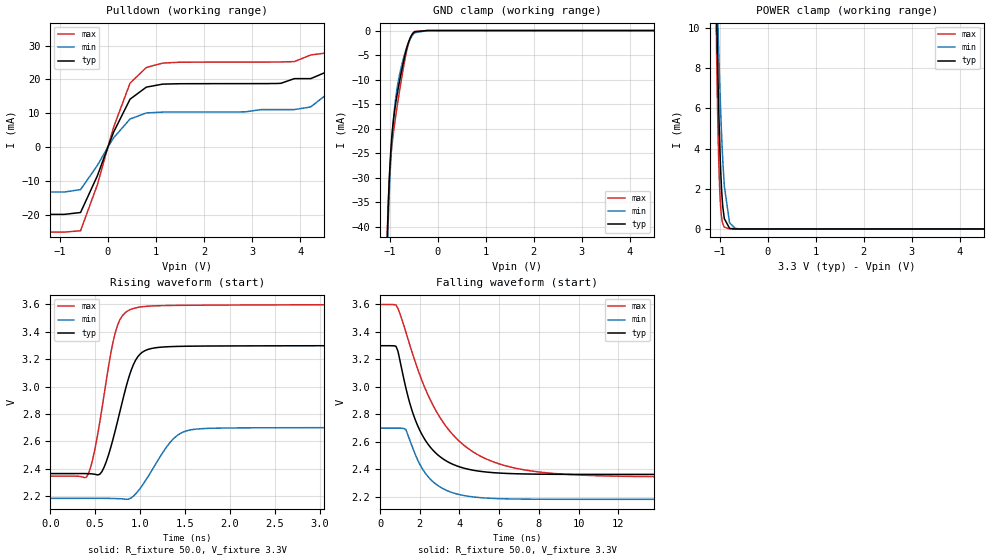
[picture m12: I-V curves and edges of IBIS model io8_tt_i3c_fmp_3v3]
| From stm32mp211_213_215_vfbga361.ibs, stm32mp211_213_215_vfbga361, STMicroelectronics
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[Model]   io8_tt_i3c_fmp_3v3
Model_type I/O_open_drain
Polarity   Non-Inverting
Enable   Active-Low
| CAP_THRESHOLD on pad IOTT is "UDTCAPC" :
| Rising=30.0% of vddiov33m   Falling=70.0% of vddiov33m
| C_comp min and max val. don't necessarily correlate with the min and max pvt
| but are the smallest and greatest pad capacitance found.
| var   typ   min   max
C_comp   1.30320pF  1.06495pF  2.26775pF
|C_comp_pulldown   1.30320pF  1.06495pF  2.26775pF
Vinl = 1.35V
Vinh = 1.8V
Vmeas = 1.65V   | Reference voltage for timing measurements
Cref  = 50.0pF   | Timing specification test load capacitance value
Rref  = 1.0MOhm   | Timing specification test load resistance value
Vref  = 1.815V   | Timing specification test load voltage
[Model Spec]
| TIME_THRESHOLD on pin ZIV08M is "CMOS" :
| Rising=50.0% of vddv08m   Falling=50.0% of vddv08m
Vinl 1.08570V 868.70000mV 1.21270V
Vinh 1.55630V 1.26330V 1.71030V
| variable   typ   min   max
[Temperature Range] 25.0 125.0 -40.0
| variable   typ   min   max
[Voltage Range] 3.3V 2.7V 3.6V
| variable   typ   min   max
[POWER Clamp Reference] 3.3V 2.7V 3.6V
| variable   typ   min   max
[GND Clamp Reference] 0V 0V 0V
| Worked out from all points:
|   slope of the pulldown table from 0 to 0.495 V, typ, clamps not added: 34.1 ohm
|   GND clamp passes 1 mA (typ) near -0.55 V on its own axis
|   POWER clamp passes 1 mA (typ) near -0.93 V on its own axis
|   rising waveform, R_fixture 50.0, V_fixture 3.3V: 20-80 % time 226ps typ, 308ps min, 195ps max; typ from 2.36 V to 3.3 V
|   falling waveform, R_fixture 50.0, V_fixture 3.3V: 20-80 % time 1.48ns typ, 1.34ns min, 2.66ns max; typ from 3.3 V to 2.36 V
[POWER Clamp]
-3.3V     1.353A     318.4mA    2.015A
-1.07V    12.07mA    13.62mA    10.38mA
-1.06V    10.79mA    12.67mA    8.742mA
-1.05V    9.57mA     11.75mA    7.25mA
-1.03V    7.34mA     9.996mA    4.745mA
-1V       4.587mA    7.593mA    2.212mA
-980mV    3.182mA    6.169mA    1.235mA
-950mV    1.703mA    4.334mA    479uA
-900mV    514.6uA    2.139mA    90.78uA
-790mV    28.73uA    299.8uA    2.713uA
-670mV    1.278uA    27.48uA    388.8nA
6.6V      0A         0A         0A
[GND Clamp]
-3.3V     -3.772A    -3.743A    -3.788A
-1.05V    -42.34mA   -45.44mA   -41.2mA
-1.04V    -38.9mA    -42mA      -37.88mA
-1.03V    -35.84mA   -38.88mA   -35.06mA
-1V       -28.57mA   -31.07mA   -28.88mA
-970mV    -23.48mA   -25.09mA   -24.97mA
-920mV    -18.07mA   -17.99mA   -20.63mA
-860mV    -13.91mA   -12.68mA   -16.46mA
-770mV    -9.031mA   -7.879mA   -10.78mA
-640mV    -3.394mA   -3.285mA   -3.897mA
-480mV    -254.3uA   -469.3uA   -191.8uA
6.6V      220.4nA    5.137uA    223.2nA
| variable   typ   min   max
[Pullup Reference] 3.3V 2.7V 3.6V
| variable   typ   min   max
[Pulldown Reference] 0V 0V 0V
[Pulldown]
-3.3V     -19.95mA   -13.34mA   -25.2mA
-570mV    -19.4mA    -12.62mA   -24.8mA
-220mV    -8.542mA   -5.471mA   -11.2mA
120mV     4.438mA    2.727mA    5.906mA
460mV     14.14mA    8.269mA    18.88mA
800mV     17.71mA    10.08mA    23.52mA
3.88V     20.22mA    11.06mA    25.27mA
4.22V     20.22mA    11.84mA    27.23mA
4.56V     22.27mA    15.63mA    27.84mA
4.9V      31.19mA    28.07mA    34.84mA
5.24V     59.66mA    64.92mA    58.18mA
6.6V      396.6mA    415.2mA    364.3mA
[Ramp]
dV/dt_r 562.25519mV/225.76963ps 311.01791mV/307.21275ps 753.53172mV/193.88812ps
dV/dt_f 562.25326mV/1.4805ns 311.01971mV/1.33977ns 753.51927mV/2.65596ns
R_load = 50.0
| Removed startup time: 0s 0s 0s  .
| Removed end time: 24.975ns.
[Rising Waveform]
R_fixture   = 50.0
V_fixture   = 3.3V
V_fixture_min = 2.7V
V_fixture_max = 3.6V
0s        2.363V     2.182V     2.344V
425ps     2.362V     2.182V     2.361V
575ps     2.377V     2.182V     2.836V
675ps     2.558V     2.181V     3.247V
750ps     2.747V     2.18V      3.45V
925ps     3.159V     2.197V     3.571V
1.075ns   3.268V     2.326V     3.587V
1.425ns   3.294V     2.647V     3.594V
1.825ns   3.296V     2.695V     3.596V
24.98ns   3.3V       2.7V       3.6V
| Removed startup time: 0s 0s 0s  .
| Removed end time: 24.9ns.
[Falling Waveform]
R_fixture   = 50.0
V_fixture   = 3.3V
V_fixture_min = 2.7V
V_fixture_max = 3.6V
0s        3.3V       2.7V       3.6V
800ps     3.296V     2.7V       3.597V
1.3ns     2.992V     2.689V     3.399V
1.7ns     2.789V     2.535V     3.213V
2.1ns     2.656V     2.412V     3.05V
2.6ns     2.55V      2.319V     2.885V
3.9ns     2.423V     2.22V      2.617V
5.8ns     2.375V     2.188V     2.45V
10.2ns    2.363V     2.182V     2.357V
24.9ns    2.363V     2.182V     2.344V
